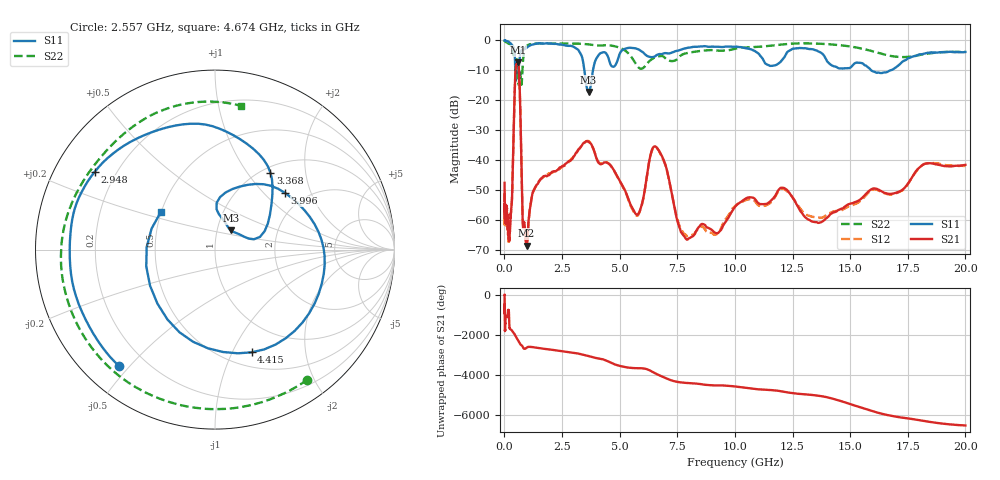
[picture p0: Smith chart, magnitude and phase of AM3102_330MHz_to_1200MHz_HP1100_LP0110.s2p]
! Date/Time: Tue, Sep 11, 2018 5:21 PM
! Network Analyzer: Agilent Technologies E8362B Rev: A.07.50.63
! Sweep from 0.010 to 20.000 GHz, 1601 Points, Sweep Type: LOG
! Power Supply: 4.949 V, 0.001 A
# Hz S DB R 50
!freq MagS11 AngS11 MagS21 AngS21 MagS12 AngS12 MagS22 AngS22
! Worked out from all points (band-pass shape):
!   1601 points, 10 MHz to 20 GHz, reference 50 ohm
!   highest |S21| = -7.25 dB at 578 MHz (marker M1); lowest = -68.4 dB at 960.9 MHz (marker M2)
!   |S21| within 3 dB of the highest: 481.2 MHz to 633.3 MHz (152.1 MHz wide, 27.3 % of centre)
!   lowest |S11| = -17.2 dB at 3.651 GHz (marker M3), VSWR 1.32, Z = 58.2 + j12.6 ohm
!   |S11| at or under -10 dB: 472.5 MHz to 521.4 MHz (48.92 MHz wide, 9.84 % of centre); 3.471 GHz to 3.842 GHz (371.1 MHz wide, 10.1 % of centre); 15.92 GHz to 16.75 GHz (837.8 MHz wide, 5.13 % of centre)
!   |S22| runs from -14.8 to -0.1 dB; largest |S21 - S12| = 0.0064
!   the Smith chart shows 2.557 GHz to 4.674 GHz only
!   S11 on the Smith chart (normalised r, x): 2.557 GHz: 0.11, -0.47; 2.948 GHz: 0.12, +0.29; 3.368 GHz: 1.09, +1.30; 3.996 GHz: 1.58, +1.34; 4.415 GHz: 0.66, -1.19; 4.674 GHz: 0.50, +0.24
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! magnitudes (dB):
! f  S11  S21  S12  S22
! 10 MHz  0.0  -47.5  -53.9  -0.1
! 35.55 MHz  -0.1  -60.4  -59.5  -0.3
! 126.4 MHz  -0.3  -58.8  -61.3  -0.8
! 207.2 MHz  -0.6  -65.9  -66.6  -1.2
! 319.2 MHz  -1.5  -54.1  -54.3  -2.6
! 447.2 MHz  -4.5  -17.1  -17.1  -4.5
! 578 MHz  -8.3  -7.2  -7.3  -10.1
! 666.5 MHz  -5.3  -16.5  -16.5  -10.9
! 798.4 MHz  -3.1  -61.0  -60.3  -7.8
! 960.9 MHz  -2.5  -68.4  -68.6  -2.0
! 1.59 GHz  -1.0  -46.1  -46.1  -1.0
! 2.557 GHz  -1.5  -41.9  -41.9  -1.0
! 2.948 GHz  -2.0  -39.5  -39.2  -1.0
! 3.368 GHz  -5.5  -34.9  -35.0  -1.2
! 3.651 GHz  -17.2  -33.8  -33.5  -1.3
! 3.996 GHz  -6.0  -39.4  -39.2  -1.7
! 4.415 GHz  -4.3  -40.7  -40.6  -1.6
! 4.674 GHz  -8.7  -42.4  -42.5  -1.8
! 5.652 GHz  -2.6  -57.3  -57.7  -7.2
! 6.549 GHz  -5.3  -35.3  -35.5  -5.6
! 7.958 GHz  -2.5  -66.3  -65.2  -4.2
! 20 GHz  -3.9  -41.5  -41.8  -3.8
